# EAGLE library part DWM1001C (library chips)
The DWM1001 module is based on Decawave's DW1000 Ultra Wideband (UWB) transceiver IC, which is an IEEE 802.15.4- 2011 UWB implementation. It integrates UWB and Bluetooth® antenna, all RF circuitry, Nordic Semiconductor nRF52832 and a motion sensor.
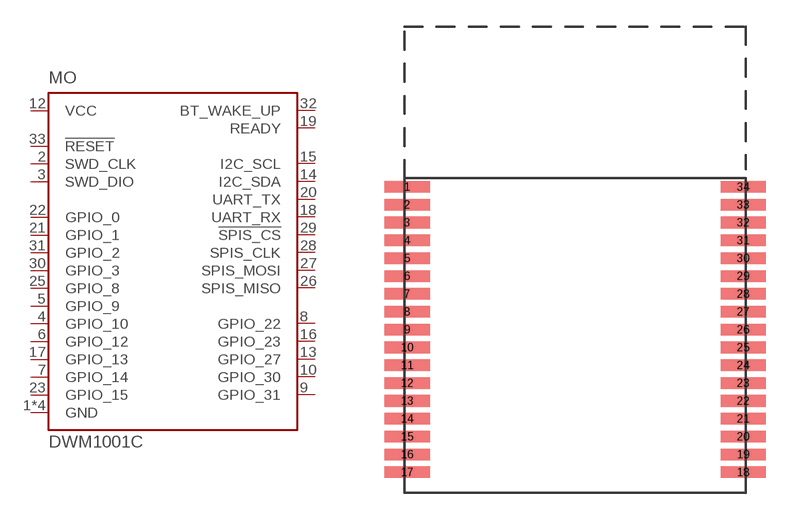
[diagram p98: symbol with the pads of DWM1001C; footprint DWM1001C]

Designator prefix MO

## DWM1001C (DIGIKEY: 1479-1004-1-ND; MPN: DWM1001C)  [DWM1001C]
1  GND
2  SWD_CLK
3  SWD_DIO
4  GPIO_10
5  GPIO_9
6  GPIO_12
7  GPIO_14
8  GPIO_22
9  GPIO_31
10  GPIO_30
11  GND
12  VCC
13  GPIO_27
14  I2C_SDA
15  I2C_SCL
16  GPIO_23
17  GPIO_13
18  UART_RX
19  READY
20  UART_TX
21  GPIO_1
22  GPIO_0
23  GPIO_15
24  GND
25  GPIO_8
26  SPIS_MISO
27  SPIS_MOSI
28  SPIS_CLK
29  !SPIS_CS
30  GPIO_3
31  GPIO_2
32  BT_WAKE_UP
33  !RESET
34  GND

## Footprint DWM1001C (pad centres in mm)
DWM1001C Castillated Footprint
smd 2.54 x 0.65: 1 -9.42,8; 2 -9.42,7; 3 -9.42,6; 4 -9.42,5; 5 -9.42,4; 6 -9.42,3; 7 -9.42,2; 8 -9.42,1; 9 -9.42,0; 10 -9.42,-1; 11 -9.42,-2; 12 -9.42,-3; 13 -9.42,-4; 14 -9.42,-5; 15 -9.42,-6; 16 -9.42,-7; 17 -9.42,-8; 18 9.42,-8; 19 9.42,-7; 20 9.42,-6; 21 9.42,-5; 22 9.42,-4; 23 9.42,-3; 24 9.42,-2; 25 9.42,-1; 26 9.42,0; 27 9.42,1; 28 9.42,2; 29 9.42,3; 30 9.42,4; 31 9.42,5; 32 9.42,6; 33 9.42,7; 34 9.42,8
